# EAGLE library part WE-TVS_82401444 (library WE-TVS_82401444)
TVS Diode Array WE-TVS, Super Speed Serie - Low capazity - No leakage current - Low clamping voltage - high ESD voltage protection -- SATA -- DisplayPort -- DVI -- HDMI
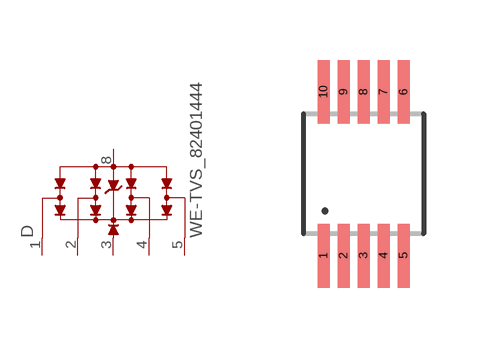
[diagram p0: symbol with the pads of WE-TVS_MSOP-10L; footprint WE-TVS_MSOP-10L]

Designator prefix D

## WE-TVS_82401444 (MPN: 82401444; OC_FARNELL: 1825863; OC_NEWARK: 79R6952; PACKAGE: MSOP-10L; SUPPLIER: Wuerth Elektronik)  [WE-TVS_MSOP-10L]
1  1  pas
2  2  pas
3  VDD  pwr
4  3  pas
5  4  pas
8  GND  pwr

## Footprint WE-TVS_MSOP-10L (pad centres in mm)
TVS Diode Array WE-TVS
smd 0.3 x 1.6: 1 -1,-2.05; 2 -0.5,-2.05; 3 0,-2.05; 4 0.5,-2.05; 5 1,-2.05; 6 1,2.05; 7 0.5,2.05; 8 0,2.05; 9 -0.5,2.05; 10 -1,2.05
